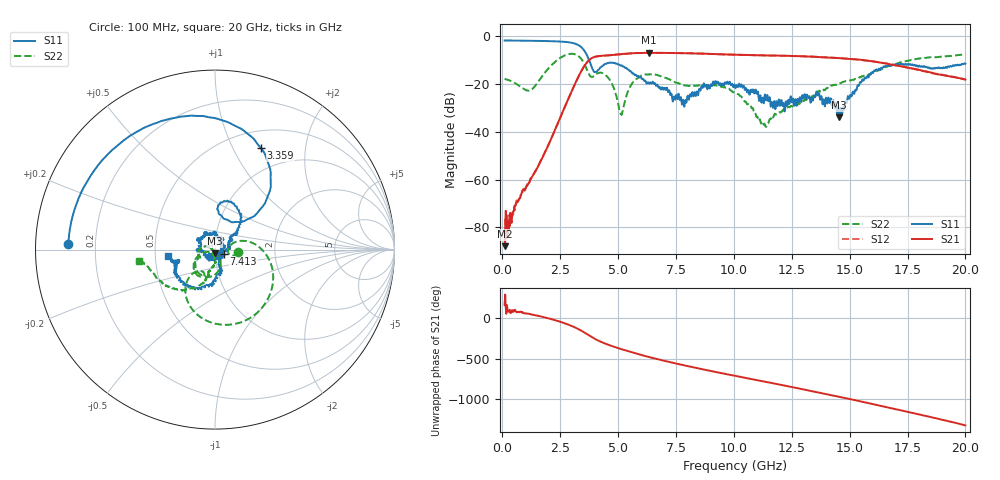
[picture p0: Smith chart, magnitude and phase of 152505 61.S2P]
!  2-Port S-parameters saved by WinCal
! VAR MeasName=S-Parameters (CALIBRATED_DATA) read from VNA (N5230C)
! VAR MeasDate=4/10/2015 9:34:59 AM
! VAR NAME=152505 61
! VAR FILENAME=152505 61.S2P
! VAR DATE=4/10/2015 9:34:59 AM
! VAR PHYS_PORTS=1,2
# Hz S DB R 50
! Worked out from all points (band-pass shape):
!   801 points, 100 MHz to 20 GHz, reference 50 ohm
!   highest |S21| = -6.91 dB at 6.319 GHz (marker M1); lowest = -87.9 dB at 100 MHz (marker M2)
!   |S21| within 3 dB of the highest: 3.753 GHz to 15.52 GHz (11.76 GHz wide, 122 % of centre)
!   lowest |S11| = -33.9 dB at 14.55 GHz (marker M3), VSWR 1.04, Z = 49.7 - j1.99 ohm
!   |S11| at or under -10 dB: 3.747 GHz to end of sweep
!   |S22| runs from -38.0 to -7.3 dB; largest |S21 - S12| = 0.0055
!   S11 on the Smith chart (normalised r, x): 100 MHz: 0.10, +0.02; 3.359 GHz: 0.70, +1.29; 7.413 GHz: 1.10, -0.05; 20 GHz: 0.58, -0.05
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1e8  -1.75 177.6  -87.89 165.2  -87.57 117.8  -17.77 -6.0
1.169625e9  -1.86 151.8  -61.06 56.6  -61.28 55.5  -22.75 -0.1
2.5875e9  -2.26 108.9  -32.11 -50.1  -32.17 -50.6  -8.55 -30.6
3.358625e9  -4.15 65.6  -15.55 -144.6  -15.58 -144.3  -8.89 -110.0
3.43325e9  -4.74 60.1  -14.21 -156.5  -14.23 -156.3  -9.75 -118.1
4.154625e9  -14.01 83.5  -8.31 82.8  -8.30 82.8  -15.32 -118.1
4.677e9  -11.11 75.0  -7.90 22.2  -7.92 22.3  -18.89 -155.9
5.12475e9  -12.24 53.4  -7.46 -20.8  -7.51 -20.7  -32.56 -120.5
5.62225e9  -15.62 40.6  -7.07 -63.9  -7.12 -64.0  -19.51 -74.9
6.31875e9  -19.65 35.4  -6.91 -118.6  -6.97 -118.6  -15.98 -114.6
6.741625e9  -21.44 29.2  -6.94 -148.9  -6.96 -149.0  -16.41 -135.3
7.41325e9  -25.22 -25.0  -6.99 165.9  -6.99 166.0  -19.10 -151.8
7.861e9  -29.51 -91.4  -7.09 136.7  -7.06 137.1  -20.53 -152.7
8.632125e9  -21.21 -173.2  -7.27 89.5  -7.26 89.4  -20.48 -155.8
1.005e10  -20.84 108.9  -7.70 6.7  -7.74 6.7  -23.92 166.4
1.136838e10  -25.58 27.7  -8.01 -67.9  -7.97 -67.6  -37.78 -148.8
1.338325e10  -25.97 -111.5  -8.56 176.4  -8.53 176.5  -24.99 -90.7
1.455238e10  -33.92 -97.0  -9.14 106.7  -9.15 106.8  -19.92 -99.9
1.554738e10  -18.07 -74.4  -9.92 44.7  -10.00 44.7  -16.68 -103.4
1.669162e10  -12.12 -116.4  -11.64 -28.3  -11.58 -28.9  -12.45 -116.2
1.848262e10  -13.56 -162.1  -15.07 -144.3  -15.20 -143.7  -8.81 -153.4
2e10  -11.47 -171.8  -18.15 110.8  -18.13 111.3  -7.38 -171.3
